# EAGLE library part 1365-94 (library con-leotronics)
DUAL ROW STRAIGHT HEADER 1364 SERIES. 1.27mm x 1.27mm. Without Fixing Post. SMT Source: http://www.leotronics.co.uk/Conexcon/Data%20Sheets/sec.%20A/1364ing.pdf
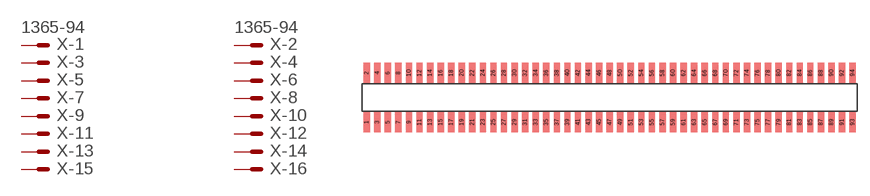
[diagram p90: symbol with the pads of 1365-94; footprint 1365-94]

Designator prefix X; gates -1=MVAL -2=MVAL -3=M -4=M -5=M -6=M -7=M -8=M -9=M -10=M -11=M -12=M -13=M -14=M -15=M -16=M -17=M -18=M -19=M -20=M -21=M -22=M -23=M -24=M -25=M -26=M -27=M -28=M -29=M -30=M -31=M -32=M -33=M -34=M -35=M -36=M -37=M -38=M -39=M -40=M -41=M -42=M -43=M -44=M -45=M -46=M -47=M -48=M -49=M -50=M -51=M -52=M -53=M -54=M -55=M -56=M -57=M -58=M -59=M -60=M -61=M -62=M -63=M -64=M -65=M -66=M -67=M -68=M -69=M -70=M -71=M -72=M -73=M -74=M -75=M -76=M -77=M -78=M -79=M -80=M -81=M -82=M -83=M -84=M -85=M -86=M -87=M -88=M -89=M -90=M -91=M -92=M -93=M -94=M

## 1365-94 (OC_FARNELL: unknown; OC_NEWARK: unknown)  [1365-94]
1  -1:S  pas
2  -2:S  pas
3  -3:S  pas
4  -4:S  pas
5  -5:S  pas
6  -6:S  pas
7  -7:S  pas
8  -8:S  pas
9  -9:S  pas
10  -10:S  pas
11  -11:S  pas
12  -12:S  pas
13  -13:S  pas
14  -14:S  pas
15  -15:S  pas
16  -16:S  pas
17  -17:S  pas
18  -18:S  pas
19  -19:S  pas
20  -20:S  pas
21  -21:S  pas
22  -22:S  pas
23  -23:S  pas
24  -24:S  pas
25  -25:S  pas
26  -26:S  pas
27  -27:S  pas
28  -28:S  pas
29  -29:S  pas
30  -30:S  pas
31  -31:S  pas
32  -32:S  pas
33  -33:S  pas
34  -34:S  pas
35  -35:S  pas
36  -36:S  pas
37  -37:S  pas
38  -38:S  pas
39  -39:S  pas
40  -40:S  pas
41  -41:S  pas
42  -42:S  pas
43  -43:S  pas
44  -44:S  pas
45  -45:S  pas
46  -46:S  pas
47  -47:S  pas
48  -48:S  pas
49  -49:S  pas
50  -50:S  pas
51  -51:S  pas
52  -52:S  pas
53  -53:S  pas
54  -54:S  pas
55  -55:S  pas
56  -56:S  pas
57  -57:S  pas
58  -58:S  pas
59  -59:S  pas
60  -60:S  pas
61  -61:S  pas
62  -62:S  pas
63  -63:S  pas
64  -64:S  pas
65  -65:S  pas
66  -66:S  pas
67  -67:S  pas
68  -68:S  pas
69  -69:S  pas
70  -70:S  pas
71  -71:S  pas
72  -72:S  pas
73  -73:S  pas
74  -74:S  pas
75  -75:S  pas
76  -76:S  pas
77  -77:S  pas
78  -78:S  pas
79  -79:S  pas
80  -80:S  pas
81  -81:S  pas
82  -82:S  pas
83  -83:S  pas
84  -84:S  pas
85  -85:S  pas
86  -86:S  pas
87  -87:S  pas
88  -88:S  pas
89  -89:S  pas
90  -90:S  pas
91  -91:S  pas
92  -92:S  pas
93  -93:S  pas
94  -94:S  pas

## Footprint 1365-94 (pad centres in mm)
DUAL ROW STRAIGHT HEADER 1364 SERIES. 1.27mm x 1.27mm. Without Fixing Post. SMT Source: http://www.leotronics.co.uk/Conexcon/Data%20Sheets/sec.%20A/1364ing.pdf
smd 0.76 x 2.4: 1 -29.21,-2.95; 2 -29.21,2.95; 3 -27.94,-2.95; 4 -27.94,2.95; 5 -26.67,-2.95; 6 -26.67,2.95; 7 -25.4,-2.95; 8 -25.4,2.95; 9 -24.13,-2.95; 10 -24.13,2.95; 11 -22.86,-2.95; 12 -22.86,2.95; 13 -21.59,-2.95; 14 -21.59,2.95; 15 -20.32,-2.95; 16 -20.32,2.95; 17 -19.05,-2.95; 18 -19.05,2.95; 19 -17.78,-2.95; 20 -17.78,2.95; 21 -16.51,-2.95; 22 -16.51,2.95; 23 -15.24,-2.95; 24 -15.24,2.95; 25 -13.97,-2.95; 26 -13.97,2.95; 27 -12.7,-2.95; 28 -12.7,2.95; 29 -11.43,-2.95; 30 -11.43,2.95; 31 -10.16,-2.95; 32 -10.16,2.95; 33 -8.89,-2.95; 34 -8.89,2.95; 35 -7.62,-2.95; 36 -7.62,2.95; 37 -6.35,-2.95; 38 -6.35,2.95; 39 -5.08,-2.95; 40 -5.08,2.95; 41 -3.81,-2.95; 42 -3.81,2.95; 43 -2.54,-2.95; 44 -2.54,2.95; 45 -1.27,-2.95; 46 -1.27,2.95; 47 0,-2.95; 48 0,2.95; 49 1.27,-2.95; 50 1.27,2.95; 51 2.54,-2.95; 52 2.54,2.95; 53 3.81,-2.95; 54 3.81,2.95; 55 5.08,-2.95; 56 5.08,2.95; 57 6.35,-2.95; 58 6.35,2.95; 59 7.62,-2.95; 60 7.62,2.95; 61 8.89,-2.95; 62 8.89,2.95; 63 10.16,-2.95; 64 10.16,2.95; 65 11.43,-2.95; 66 11.43,2.95; 67 12.7,-2.95; 68 12.7,2.95; 69 13.97,-2.95; 70 13.97,2.95; 71 15.24,-2.95; 72 15.24,2.95; 73 16.51,-2.95; 74 16.51,2.95; 75 17.78,-2.95; 76 17.78,2.95; 77 19.05,-2.95; 78 19.05,2.95; 79 20.32,-2.95; 80 20.32,2.95; 81 21.59,-2.95; 82 21.59,2.95; 83 22.86,-2.95; 84 22.86,2.95; 85 24.13,-2.95; 86 24.13,2.95; 87 25.4,-2.95; 88 25.4,2.95; 89 26.67,-2.95; 90 26.67,2.95; 91 27.94,-2.95; 92 27.94,2.95; 93 29.21,-2.95; 94 29.21,2.95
